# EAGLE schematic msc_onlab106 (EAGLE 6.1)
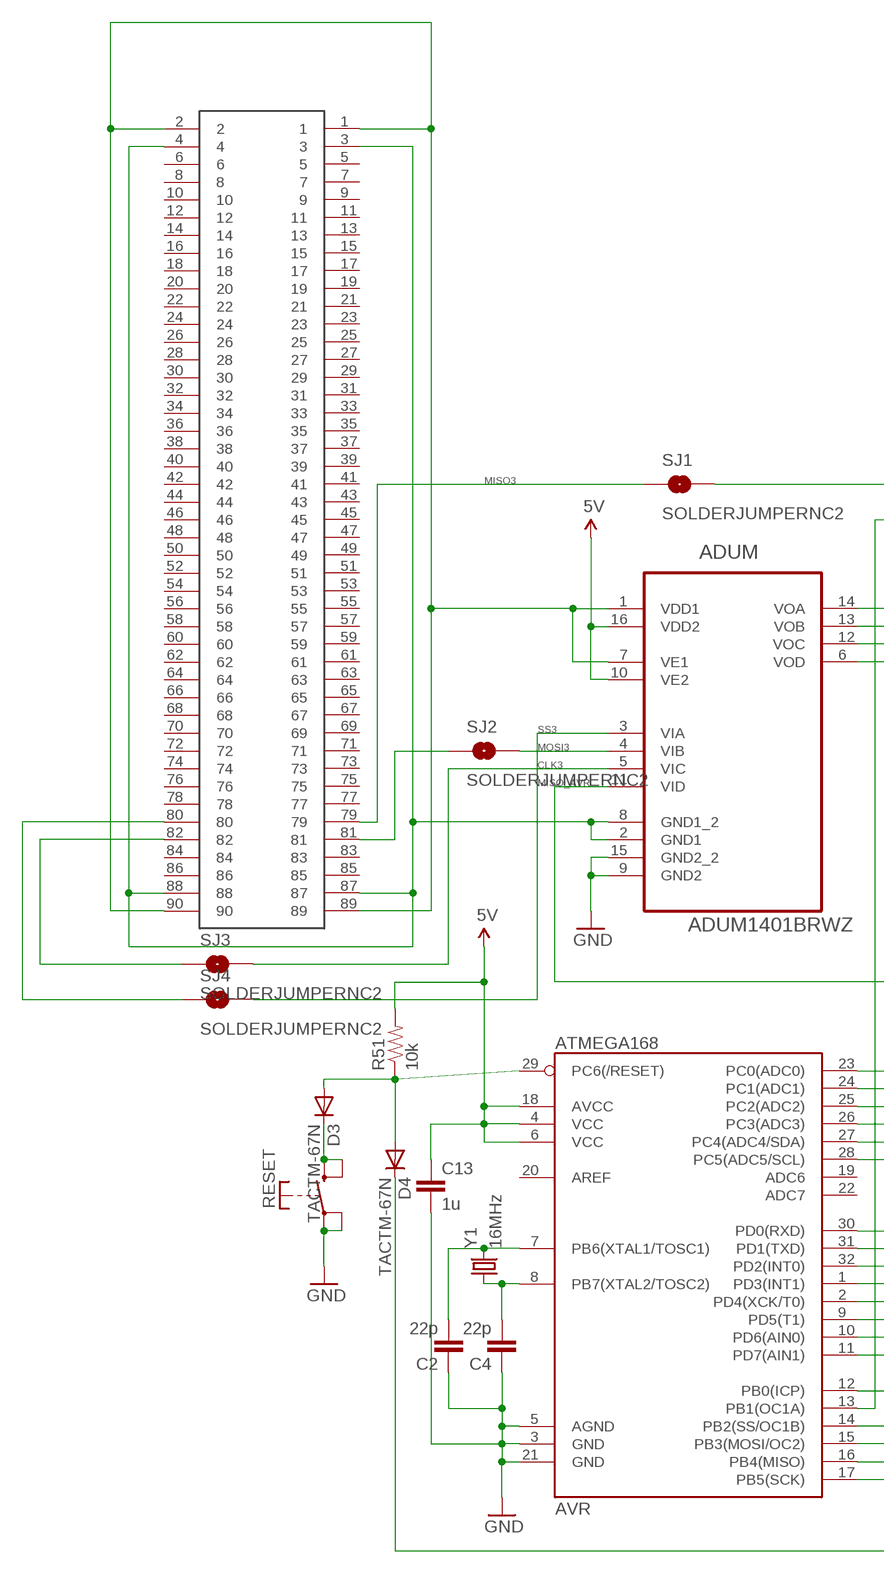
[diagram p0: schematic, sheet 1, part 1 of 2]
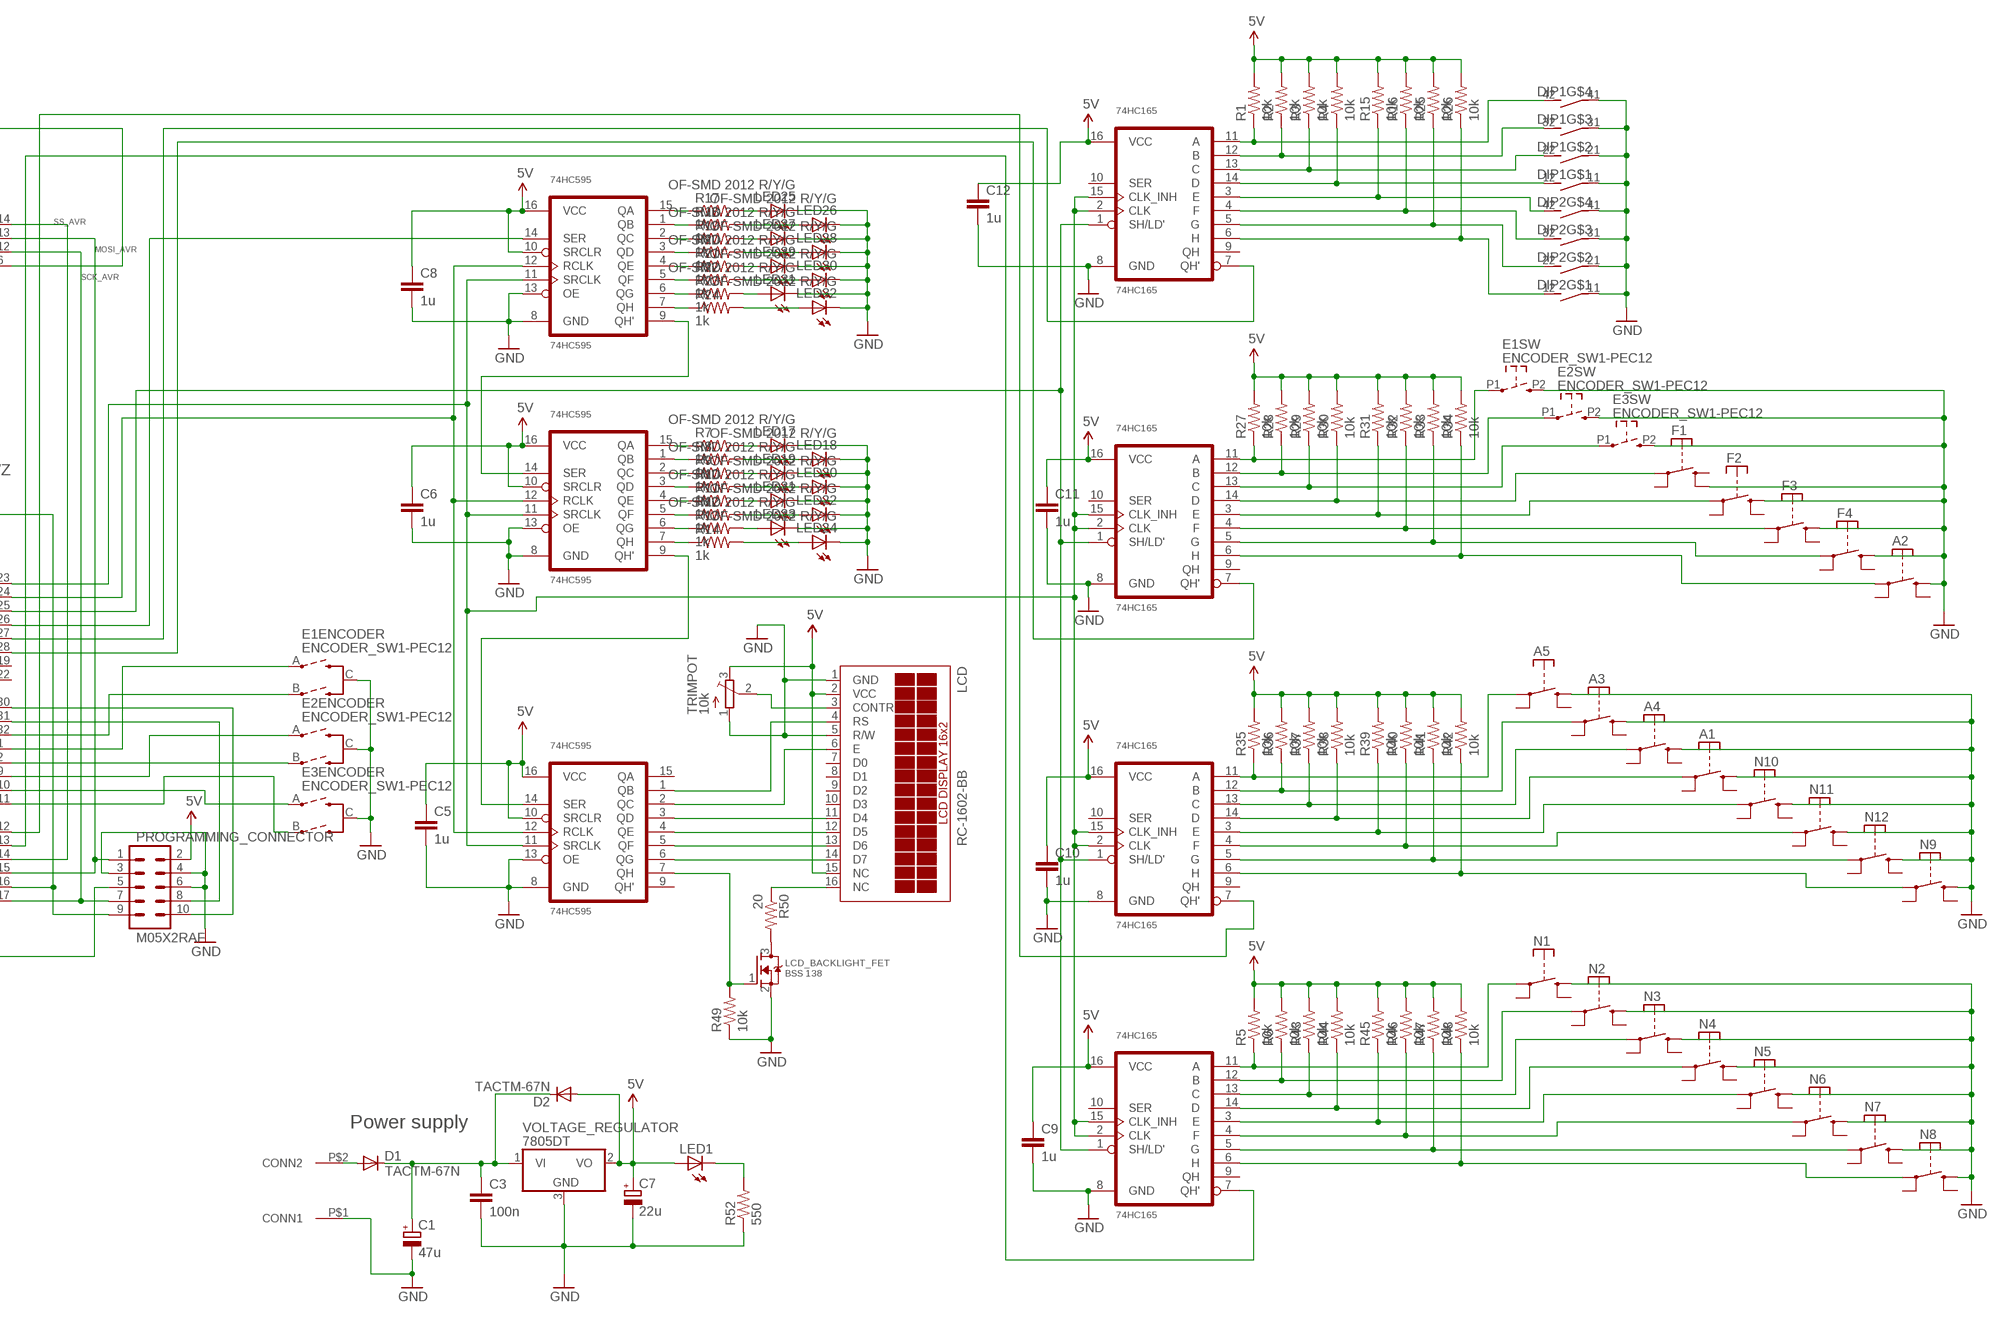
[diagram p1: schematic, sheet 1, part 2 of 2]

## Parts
A1  TACTM-67N  BUTTON_SMD  [SMD]
A2  TACTM-67N  BUTTON_SMD  [SMD]
A3  TACTM-67N  BUTTON_SMD  [SMD]
A4  TACTM-67N  BUTTON_SMD  [SMD]
A5  TACTM-67N  BUTTON_SMD  [SMD]
ADUM  ADUM1401BRWZ  [SOIC127P1032X265-16N]
AVR  ATMEGA168  [TQFP32-08]
C1  47u  CPOL-EUD/7343-31W  [D/7343-31W]
C2  22p  CAP0603-CAP  [0603-CAP]
C3  100n  C-EUC0805K  [C0805K]
C4  22p  CAP0603-CAP  [0603-CAP]
C5  1u  CAP0603-CAP  [0603-CAP]
C6  1u  CAP0603-CAP  [0603-CAP]
C7  22u  CPOL-EUSMCB  [SMC_B]
C8  1u  CAP0603-CAP  [0603-CAP]
C9  1u  CAP0603-CAP  [0603-CAP]
C10  1u  CAP0603-CAP  [0603-CAP]
C11  1u  CAP0603-CAP  [0603-CAP]
C12  1u  CAP0603-CAP  [0603-CAP]
C13  1u  CAP0603-CAP  [0603-CAP]
CONNECTOR  SAMTEC_TFC  [SAMTEC-TFC]
D1  TACTM-67N  DIODESMA-ALT  [SMA-DIODE_ALT]
D2  TACTM-67N  DIODESMA-ALT  [SMA-DIODE_ALT]
D3  TACTM-67N  DIODESMA-ALT  [SMA-DIODE_ALT]
D4  TACTM-67N  DIODESMA-ALT  [SMA-DIODE_ALT]
DIP1  DIP04PIANO  [DIP04PIANO]
DIP2  DIP04PIANO  [DIP04PIANO]
E1  ENCODER_SW1-PEC12  [PEC12_INCREMENTAL_ENCODER]
E2  ENCODER_SW1-PEC12  [PEC12_INCREMENTAL_ENCODER]
E3  ENCODER_SW1-PEC12  [PEC12_INCREMENTAL_ENCODER]
F1  TACTM-67N  BUTTON_SMD  [SMD]
F2  TACTM-67N  BUTTON_SMD  [SMD]
F3  TACTM-67N  BUTTON_SMD  [SMD]
F4  TACTM-67N  BUTTON_SMD  [SMD]
IN_1  74HC165  [TI_PW]
IN_2  74HC165  [TI_PW]
IN_3  74HC165  [TI_PW]
IN_4  74HC165  [TI_PW]
LCD  RC-1602-BB  TUXGR_16X2_R2  [TUXGR_16X2_R2]
LCD_BACKLIGHT_FET  BSS 138  MOSFET-NREFLOW  [SOT23]
LED1  LEDCHIPLED_0805  [CHIPLED_0805]
LED17  OF-SMD 2012 R/Y/G  LEDCHIPLED_0805  [CHIPLED_0805]
LED18  OF-SMD 2012 R/Y/G  LEDCHIPLED_0805  [CHIPLED_0805]
LED19  OF-SMD 2012 R/Y/G  LEDCHIPLED_0805  [CHIPLED_0805]
LED20  OF-SMD 2012 R/Y/G  LEDCHIPLED_0805  [CHIPLED_0805]
LED21  OF-SMD 2012 R/Y/G  LEDCHIPLED_0805  [CHIPLED_0805]
LED22  OF-SMD 2012 R/Y/G  LEDCHIPLED_0805  [CHIPLED_0805]
LED23  OF-SMD 2012 R/Y/G  LEDCHIPLED_0805  [CHIPLED_0805]
LED24  OF-SMD 2012 R/Y/G  LEDCHIPLED_0805  [CHIPLED_0805]
LED25  OF-SMD 2012 R/Y/G  LEDCHIPLED_0805  [CHIPLED_0805]
LED26  OF-SMD 2012 R/Y/G  LEDCHIPLED_0805  [CHIPLED_0805]
LED27  OF-SMD 2012 R/Y/G  LEDCHIPLED_0805  [CHIPLED_0805]
LED28  OF-SMD 2012 R/Y/G  LEDCHIPLED_0805  [CHIPLED_0805]
LED29  OF-SMD 2012 R/Y/G  LEDCHIPLED_0805  [CHIPLED_0805]
LED30  OF-SMD 2012 R/Y/G  LEDCHIPLED_0805  [CHIPLED_0805]
LED31  OF-SMD 2012 R/Y/G  LEDCHIPLED_0805  [CHIPLED_0805]
LED32  OF-SMD 2012 R/Y/G  LEDCHIPLED_0805  [CHIPLED_0805]
N1  TACTM-67N  BUTTON_SMD  [SMD]
N2  TACTM-67N  BUTTON_SMD  [SMD]
N3  TACTM-67N  BUTTON_SMD  [SMD]
N4  TACTM-67N  BUTTON_SMD  [SMD]
N5  TACTM-67N  BUTTON_SMD  [SMD]
N6  TACTM-67N  BUTTON_SMD  [SMD]
N7  TACTM-67N  BUTTON_SMD  [SMD]
N8  TACTM-67N  BUTTON_SMD  [SMD]
N9  TACTM-67N  BUTTON_SMD  [SMD]
N10  TACTM-67N  BUTTON_SMD  [SMD]
N11  TACTM-67N  BUTTON_SMD  [SMD]
N12  TACTM-67N  BUTTON_SMD  [SMD]
POWER_CONNECTOR  NSL39_2_CONNECTOR  [NSL39_2_CONNECTOR]
PROGRAMMING_CONNECTOR  M05X2RAF  [2X5-RAF]
R1  10k  RESISTOR0603-RES  [0603-RES]
R2  10k  RESISTOR0603-RES  [0603-RES]
R3  10k  RESISTOR0603-RES  [0603-RES]
R4  10k  RESISTOR0603-RES  [0603-RES]
R5  10k  RESISTOR0603-RES  [0603-RES]
R6  10k  RESISTOR0603-RES  [0603-RES]
R7  1k  RESISTOR0603-RES  [0603-RES]
R8  1k  RESISTOR0603-RES  [0603-RES]
R9  1k  RESISTOR0603-RES  [0603-RES]
R10  1k  RESISTOR0603-RES  [0603-RES]
R11  1k  RESISTOR0603-RES  [0603-RES]
R12  1k  RESISTOR0603-RES  [0603-RES]
R13  1k  RESISTOR0603-RES  [0603-RES]
R14  1k  RESISTOR0603-RES  [0603-RES]
R15  10k  RESISTOR0603-RES  [0603-RES]
R16  10k  RESISTOR0603-RES  [0603-RES]
R17  1k  RESISTOR0603-RES  [0603-RES]
R18  1k  RESISTOR0603-RES  [0603-RES]
R19  1k  RESISTOR0603-RES  [0603-RES]
R20  1k  RESISTOR0603-RES  [0603-RES]
R21  1k  RESISTOR0603-RES  [0603-RES]
R22  1k  RESISTOR0603-RES  [0603-RES]
R23  1k  RESISTOR0603-RES  [0603-RES]
R24  1k  RESISTOR0603-RES  [0603-RES]
R25  10k  RESISTOR0603-RES  [0603-RES]
R26  10k  RESISTOR0603-RES  [0603-RES]
R27  10k  RESISTOR0603-RES  [0603-RES]
R28  10k  RESISTOR0603-RES  [0603-RES]
R29  10k  RESISTOR0603-RES  [0603-RES]
R30  10k  RESISTOR0603-RES  [0603-RES]
R31  10k  RESISTOR0603-RES  [0603-RES]
R32  10k  RESISTOR0603-RES  [0603-RES]
R33  10k  RESISTOR0603-RES  [0603-RES]
R34  10k  RESISTOR0603-RES  [0603-RES]
R35  10k  RESISTOR0603-RES  [0603-RES]
R36  10k  RESISTOR0603-RES  [0603-RES]
R37  10k  RESISTOR0603-RES  [0603-RES]
R38  10k  RESISTOR0603-RES  [0603-RES]
R39  10k  RESISTOR0603-RES  [0603-RES]
R40  10k  RESISTOR0603-RES  [0603-RES]
R41  10k  RESISTOR0603-RES  [0603-RES]
R42  10k  RESISTOR0603-RES  [0603-RES]
R43  10k  RESISTOR0603-RES  [0603-RES]
R44  10k  RESISTOR0603-RES  [0603-RES]
R45  10k  RESISTOR0603-RES  [0603-RES]
R46  10k  RESISTOR0603-RES  [0603-RES]
R47  10k  RESISTOR0603-RES  [0603-RES]
R48  10k  RESISTOR0603-RES  [0603-RES]
R49  10k  RESISTOR0603-RES  [0603-RES]
R50  20  RESISTOR0603-RES  [0603-RES]
R51  10k  RESISTOR0603-RES  [0603-RES]
R52  550  RESISTOR0603-RES  [0603-RES]
RESET  NSG 39-2  BUTTON_SMD  [SMD]
SJ1  SOLDERJUMPERNC2  [SJ_2S-NOTRACE]
SJ2  SOLDERJUMPERNC2  [SJ_2S-NOTRACE]
SJ3  SOLDERJUMPERNC2  [SJ_2S-NOTRACE]
SJ4  SOLDERJUMPERNC2  [SJ_2S-NOTRACE]
SR_OUT1  74HC595  [TI_PW]
SR_OUT2  74HC595  [TI_PW]
SR_OUT3  74HC595  [TI_PW]
TRIMPOT  10k  TRIMPOTTC33X  [TC33X]
VOLTAGE_REGULATOR  7805DT  [TO252]
Y1  16MHz  CRYSTALSMD  [HC49UP]

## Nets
3V3: ADUM.1(VDD1) ADUM.7(VE1) CONNECTOR.1 CONNECTOR.2 CONNECTOR.89 CONNECTOR.90
3V3_GND: ADUM.2(GND1) ADUM.8(GND1_2) CONNECTOR.3 CONNECTOR.4 CONNECTOR.87 CONNECTOR.88
5V: ADUM.10(VE2) ADUM.16(VDD2) AVR.4(VCC) AVR.6(VCC) AVR.18(AVCC) C5.1 C6.1 C7.+ C8.1 C9.1 C10.1 C11.1 C12.1 C13.1 D2.A IN_1.16(VCC) IN_2.16(VCC) IN_3.16(VCC) IN_4.16(VCC) LCD.2(VCC) LCD.15(NC) LED1.A PROGRAMMING_CONNECTOR.2 R1.2 R2.2 R3.2 R4.2 R5.2 R6.2 R15.2 R16.2 R25.2 R26.2 R27.2 R28.2 R29.2 R30.2 R31.2 R32.2 R33.2 R34.2 R35.2 R36.2 R37.2 R38.2 R39.2 R40.2 R41.2 R42.2 R43.2 R44.2 R45.2 R46.2 R47.2 R48.2 R51.2 SR_OUT1.10(SRCLR) SR_OUT1.16(VCC) SR_OUT2.10(SRCLR) SR_OUT2.16(VCC) SR_OUT3.10(SRCLR) SR_OUT3.16(VCC) TRIMPOT.3(E) VOLTAGE_REGULATOR.2(VO)
CLK3: ADUM.5(VIC) SJ3.2
GND: A1.P$4(P) A2.P$4(P) A3.P$4(P) A4.P$4(P) A5.P$4(P) ADUM.9(GND2) ADUM.15(GND2_2) AVR.3(GND) AVR.5(AGND) AVR.21(GND) C1.- C2.1 C3.2 C4.1 C5.2 C6.2 C7.- C8.2 C9.2 C10.2 C11.2 C12.2 C13.2 DIP1.11 DIP1.21 DIP1.31 DIP1.41 DIP2.11 DIP2.21 DIP2.31 DIP2.41 E1.C(ENCODER:C) E1.P2 E2.C(ENCODER:C) E2.P2 E3.C(ENCODER:C) E3.P2 F1.P$3(P) F2.P$4(P) F3.P$4(P) F4.P$4(P) IN_1.8(GND) IN_2.8(GND) IN_3.8(GND) IN_4.8(GND) LCD.1(GND) LCD.5(R/W) LCD_BACKLIGHT_FET.2(S) LED17.C LED18.C LED19.C LED20.C LED21.C LED22.C LED23.C LED24.C LED25.C LED26.C LED27.C LED28.C LED29.C LED30.C LED31.C LED32.C N1.P$4(P) N2.P$4(P) N3.P$4(P) N4.P$4(P) N5.P$4(P) N6.P$4(P) N7.P$4(P) N8.P$4(P) N9.P$4(P) N10.P$4(P) N11.P$4(P) N12.P$4(P) POWER_CONNECTOR.P$1(CONN1) PROGRAMMING_CONNECTOR.3 PROGRAMMING_CONNECTOR.4 PROGRAMMING_CONNECTOR.6 R49.1 R52.1 RESET.P$1(P) RESET.P$2(P) SR_OUT1.8(GND) SR_OUT1.13(OE) SR_OUT2.8(GND) SR_OUT2.13(OE) SR_OUT3.8(GND) SR_OUT3.13(OE) TRIMPOT.1(A) VOLTAGE_REGULATOR.3(GND)
IN1A: DIP1.42 IN_1.11(A) R1.1
IN1B: DIP1.32 IN_1.12(B) R2.1
IN1C: DIP1.22 IN_1.13(C) R3.1
IN1D: DIP1.12 IN_1.14(D) R4.1
IN1E: DIP2.42 IN_1.3(E) R15.1
IN1F: DIP2.32 IN_1.4(F) R16.1
IN1G: DIP2.22 IN_1.5(G) R25.1
IN1H: DIP2.12 IN_1.6(H) R26.1
IN2A: E1.P1 IN_2.11(A) R27.1
IN2B: E2.P1 IN_2.12(B) R28.1
IN2C: E3.P1 IN_2.13(C) R29.1
IN2D: F1.P$2(P) IN_2.14(D) R30.1
IN2E: F2.P$2(P) IN_2.3(E) R31.1
IN2F: F3.P$2(P) IN_2.4(F) R32.1
IN2G: F4.P$2(P) IN_2.5(G) R33.1
IN2H: A2.P$2(P) IN_2.6(H) R34.1
IN3C: A4.P$2(P) IN_3.13(C) R37.1
IN3D: A1.P$2(P) IN_3.14(D) R38.1
IN3E: IN_3.3(E) N10.P$2(P) R39.1
IN3F: IN_3.4(F) N11.P$2(P) R40.1
IN3G: IN_3.5(G) N12.P$2(P) R41.1
IN3H: IN_3.6(H) N9.P$2(P) R42.1
IN4A: IN_4.11(A) N1.P$2(P) R5.1
IN4B: IN_4.12(B) N2.P$2(P) R6.1
IN4C: IN_4.13(C) N3.P$2(P) R43.1
IN4D: IN_4.14(D) N4.P$2(P) R44.1
IN4E: IN_4.3(E) N5.P$2(P) R45.1
IN4F: IN_4.4(F) N6.P$2(P) R46.1
IN4G: IN_4.5(G) N7.P$2(P) R47.1
IN4H: IN_4.6(H) N8.P$2(P) R48.1
IN_1: AVR.27(PC4(ADC4/SDA)) IN_1.7(QH')
IN_2: AVR.28(PC5(ADC5/SCL)) IN_2.7(QH')
IN_3: AVR.12(PB0(ICP)) IN_3.7(QH')
IN_4: AVR.13(PB1(OC1A)) IN_4.7(QH')
IN_LOAD: AVR.25(PC2(ADC2)) IN_1.1(SH/LD') IN_2.1(SH/LD') IN_3.1(SH/LD') IN_4.1(SH/LD')
IO_CLK: AVR.23(PC0(ADC0)) IN_1.2(CLK) IN_1.15(CLK_INH) IN_2.2(CLK) IN_2.15(CLK_INH) IN_3.2(CLK) IN_3.15(CLK_INH) IN_4.2(CLK) IN_4.15(CLK_INH) SR_OUT1.11(SRCLK) SR_OUT2.11(SRCLK) SR_OUT3.11(SRCLK)
MISO3: CONNECTOR.79 SJ1.1
MISO_AVR: ADUM.11(VID) AVR.16(PB4(MISO)) PROGRAMMING_CONNECTOR.9
MOSI3: CONNECTOR.81 SJ2.1
MOSI_AVR: ADUM.13(VOB) AVR.15(PB3(MOSI/OC2)) PROGRAMMING_CONNECTOR.1
N$1: A5.P$2(P) IN_3.11(A) R35.1
N$2: A3.P$2(P) IN_3.12(B) R36.1
N$3: LCD.14(D7) SR_OUT1.6(QG)
N$4: LCD.13(D6) SR_OUT1.5(QF)
N$5: LCD.3(CONTR) TRIMPOT.2(S)
N$6: LCD_BACKLIGHT_FET.1(G) R49.2 SR_OUT1.7(QH)
N$7: LCD_BACKLIGHT_FET.3(D) R50.2
N$8: LCD.16(NC) R50.1
N$9: LCD.12(D5) SR_OUT1.4(QE)
N$10: LCD.11(D4) SR_OUT1.3(QD)
N$11: LCD.6(E) SR_OUT1.2(QC)
N$12: D1.A POWER_CONNECTOR.P$2(CONN2)
N$13: LCD.4(RS) SR_OUT1.1(QB)
N$14: C1.+ C3.1 D1.C D2.C VOLTAGE_REGULATOR.1(VI)
N$17: AVR.32(PD2(INT0)) E1.B(ENCODER:B)
N$20: AVR.8(PB7(XTAL2/TOSC2)) C4.2 Y1.1
N$21: CONNECTOR.82 SJ3.1
N$22: CONNECTOR.80 SJ4.1
N$23: AVR.7(PB6(XTAL1/TOSC1)) C2.2 Y1.2
N$24: AVR.1(PD3(INT1)) E1.A(ENCODER:A)
N$25: AVR.2(PD4(XCK/T0)) E2.B(ENCODER:B)
N$27: AVR.9(PD5(T1)) E2.A(ENCODER:A)
N$28: LED1.C R52.2
N$29: ADUM.4(VIB) SJ2.2
N$30: AVR.10(PD6(AIN0)) E3.A(ENCODER:A)
N$31: ADUM.6(VOD) SJ1.2
N$32: AVR.11(PD7(AIN1)) E3.B(ENCODER:B)
N$33: R7.1 SR_OUT2.15(QA)
N$34: R8.1 SR_OUT2.1(QB)
N$35: R9.1 SR_OUT2.2(QC)
N$36: R10.1 SR_OUT2.3(QD)
N$37: R11.1 SR_OUT2.4(QE)
N$38: R12.1 SR_OUT2.5(QF)
N$39: R13.1 SR_OUT2.6(QG)
N$40: R14.1 SR_OUT2.7(QH)
N$41: LED17.A R7.2
N$42: LED18.A R8.2
N$43: LED19.A R9.2
N$44: LED20.A R10.2
N$45: LED21.A R11.2
N$46: LED22.A R12.2
N$47: LED23.A R13.2
N$48: LED24.A R14.2
N$49: R17.1 SR_OUT3.15(QA)
N$50: R18.1 SR_OUT3.1(QB)
N$51: R19.1 SR_OUT3.2(QC)
N$52: R20.1 SR_OUT3.3(QD)
N$53: R21.1 SR_OUT3.4(QE)
N$54: R22.1 SR_OUT3.5(QF)
N$55: R23.1 SR_OUT3.6(QG)
N$56: R24.1 SR_OUT3.7(QH)
N$57: LED25.A R17.2
N$58: LED26.A R18.2
N$59: LED27.A R19.2
N$60: LED28.A R20.2
N$61: LED29.A R21.2
N$62: LED30.A R22.2
N$63: LED31.A R23.2
N$64: LED32.A R24.2
N$65: AVR.29(PC6(/RESET)) D3.A D4.A R51.1
N$67: D3.C RESET.P$3(P) RESET.P$4(P)
OUT: AVR.26(PC3(ADC3)) SR_OUT3.14(SER)
OUT_DAISY: SR_OUT2.14(SER) SR_OUT3.9(QH')
OUT_DAISY2: SR_OUT1.14(SER) SR_OUT2.9(QH')
OUT_LATCH: AVR.24(PC1(ADC1)) SR_OUT1.12(RCLK) SR_OUT2.12(RCLK) SR_OUT3.12(RCLK)
RESET: D4.C PROGRAMMING_CONNECTOR.5
RX: AVR.30(PD0(RXD)) PROGRAMMING_CONNECTOR.10
SCK_AVR: ADUM.12(VOC) AVR.17(PB5(SCK)) PROGRAMMING_CONNECTOR.7
SS3: ADUM.3(VIA) SJ4.2
SS_AVR: ADUM.14(VOA) AVR.14(PB2(SS/OC1B))
TX: AVR.31(PD1(TXD)) PROGRAMMING_CONNECTOR.8
Unconnected: A1.P$1(P) A1.P$3(P) A2.P$1(P) A2.P$3(P) A3.P$1(P) A3.P$3(P) A4.P$1(P) A4.P$3(P) A5.P$1(P) A5.P$3(P) AVR.19(ADC6) AVR.20(AREF) AVR.22(ADC7) CONNECTOR.5 CONNECTOR.6 CONNECTOR.7 CONNECTOR.8 CONNECTOR.9 CONNECTOR.10 CONNECTOR.11 CONNECTOR.12 CONNECTOR.13 CONNECTOR.14 CONNECTOR.15 CONNECTOR.16 CONNECTOR.17 CONNECTOR.18 CONNECTOR.19 CONNECTOR.20 CONNECTOR.21 CONNECTOR.22 CONNECTOR.23 CONNECTOR.24 CONNECTOR.25 CONNECTOR.26 CONNECTOR.27 CONNECTOR.28 CONNECTOR.29 CONNECTOR.30 CONNECTOR.31 CONNECTOR.32 CONNECTOR.33 CONNECTOR.34 CONNECTOR.35 CONNECTOR.36 CONNECTOR.37 CONNECTOR.38 CONNECTOR.39 CONNECTOR.40 CONNECTOR.41 CONNECTOR.42 CONNECTOR.43 CONNECTOR.44 CONNECTOR.45 CONNECTOR.46 CONNECTOR.47 CONNECTOR.48 CONNECTOR.49 CONNECTOR.50 CONNECTOR.51 CONNECTOR.52 CONNECTOR.53 CONNECTOR.54 CONNECTOR.55 CONNECTOR.56 CONNECTOR.57 CONNECTOR.58 CONNECTOR.59 CONNECTOR.60 CONNECTOR.61 CONNECTOR.62 CONNECTOR.63 CONNECTOR.64 CONNECTOR.65 CONNECTOR.66 CONNECTOR.67 CONNECTOR.68 CONNECTOR.69 CONNECTOR.70 CONNECTOR.71 CONNECTOR.72 CONNECTOR.73 CONNECTOR.74 CONNECTOR.75 CONNECTOR.76 CONNECTOR.77 CONNECTOR.78 CONNECTOR.83 CONNECTOR.84 CONNECTOR.85 CONNECTOR.86 F1.P$1(P) F1.P$4(P) F2.P$1(P) F2.P$3(P) F3.P$1(P) F3.P$3(P) F4.P$1(P) F4.P$3(P) IN_1.9(QH) IN_1.10(SER) IN_2.9(QH) IN_2.10(SER) IN_3.9(QH) IN_3.10(SER) IN_4.9(QH) IN_4.10(SER) LCD.7(D0) LCD.8(D1) LCD.9(D2) LCD.10(D3) N1.P$1(P) N1.P$3(P) N2.P$1(P) N2.P$3(P) N3.P$1(P) N3.P$3(P) N4.P$1(P) N4.P$3(P) N5.P$1(P) N5.P$3(P) N6.P$1(P) N6.P$3(P) N7.P$1(P) N7.P$3(P) N8.P$1(P) N8.P$3(P) N9.P$1(P) N9.P$3(P) N10.P$1(P) N10.P$3(P) N11.P$1(P) N11.P$3(P) N12.P$1(P) N12.P$3(P) SR_OUT1.9(QH') SR_OUT1.15(QA)

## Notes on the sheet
- Power supply

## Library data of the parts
A1-A5 F1-F4 N1-N12 RESET = stibi:BUTTON
ADUM = Analog Devices_By_element14_Batch_1:ADUM1401BRWZ: Quad-Channel Digital Isolators; MPN: ADUM1401BRWZ; OC_FARNELL: 1226221; OC_NEWARK: 59K3278; PACKAGE: SOIC-16; SUPPLIER: Analog Devices
AVR = SparkFun:ATMEGA168
C1 = resistor:CPOL-EU: POLARIZED CAPACITOR, European symbol
C2 C4-C6 C8-C13 = SparkFun:CAP: Capacitor
C3 = rcl:C-EU: CAPACITOR, European symbol
C7 = rcl:CPOL-EU: POLARIZED CAPACITOR, European symbol
CONNECTOR = stibi:SAMTEC_TFC
D1-D4 = SparkFun:DIODE: Diode
DIP1 DIP2 = stibi:DIP04PIANO
E1-E3 = dp_devices:ENCODER_SW1: Incremental Encoder with push switch
IN_1-IN_4 = stibi:74HC165
LCD = display-lcd:TUXGR_16X2_R2: Tuxgraphics LCD display 16x2 characters reflective, without background light Source: tuxgr_12x2_r2.pdf; OC_FARNELL: unknown; OC_NEWARK: unknown
LCD_BACKLIGHT_FET = adafruit:MOSFET-N: N-Channel Mosfet 2N7002E - 60V 260mA SOT23 [Digikey: 2N7002ET1GOSTR-ND] - REEL BSH103 - 30V 850mA SOT23 [Digikey: 568-5013-1-ND]
LED1 LED17-LED32 = adafruit:LED: LED
POWER_CONNECTOR = stibi:NSL39_2_CONNECTOR
PROGRAMMING_CONNECTOR = SparkFun:M05X2: Header 5x2 Standard 10-pin dual row 0.1" header. Commonly used with AVR-ISP. Use with Spark Fun Electronics SKU: PRT-00778
R1-R52 = SparkFun:RESISTOR: Resistor
SJ1-SJ4 = SparkFun:SOLDERJUMPER: Solder Jumper
SR_OUT1-SR_OUT3 = stibi:74HC595
TRIMPOT = adafruit:TRIMPOT: SMT trimmer potentiometer part number TC33X http://www.ladyada.net/library/eagle
VOLTAGE_REGULATOR = linear:78*: Positive VOLTAGE REGULATOR Source: http://cache.national.com/ds/LM/LM78L05.pdf http://www.fairchildsemi.com/ds/LM/LM7805.pdf
Y1 = SparkFun:CRYSTAL: Crystals

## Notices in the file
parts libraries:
SparkFun: Licensing: CC v3.0 Share-Alike You are welcome to use this library for commercial purposes.
